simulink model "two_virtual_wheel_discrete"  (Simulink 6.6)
settings: Solver=FixedStepDiscrete  SolverMode=MultiTasking  StartTime=0.0  StopTime=tfinal  RelTol=1e-3
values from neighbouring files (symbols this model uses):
  b1 = T1*k1    (= 0.15)    [two_virtual_wheel_params.m]    (also in two_virtual_wheels.m)
  b2 = T2*k2    (= 0.015)    [two_virtual_wheel_params.m]    (also in two_virtual_wheels.m)
  Jw1 = .5*1.5/4    (= 0.1875)    [two_virtual_wheel_params.m]    (also in two_virtual_wheels.m)
  Jw2 = .5*.015/4    (= 0.001875)    [two_virtual_wheel_params.m]    (also in two_virtual_wheels.m)
  k1 = .5*15    (= 7.5)    [two_virtual_wheel_params.m]    (also in two_virtual_wheels.m)
  k2 = .5*15    (= 7.5)    [two_virtual_wheel_params.m]    (also in two_virtual_wheels.m)
  step_time = 1    [two_virtual_wheel_params.m]    (also in two_virtual_wheels.m)
  T1 = 1/50    (= 0.02)    [two_virtual_wheel_params.m]    (also in two_virtual_wheels.m)
  T2 = 1/500    (= 0.002)    [two_virtual_wheel_params.m]    (also in two_virtual_wheels.m)
  Theta_z_0 = 45    [two_virtual_wheel_params.m]    (also in two_virtual_wheels.m)
undefined symbols (not defined in the file or in its folder): DiscIntNeverNeededParam

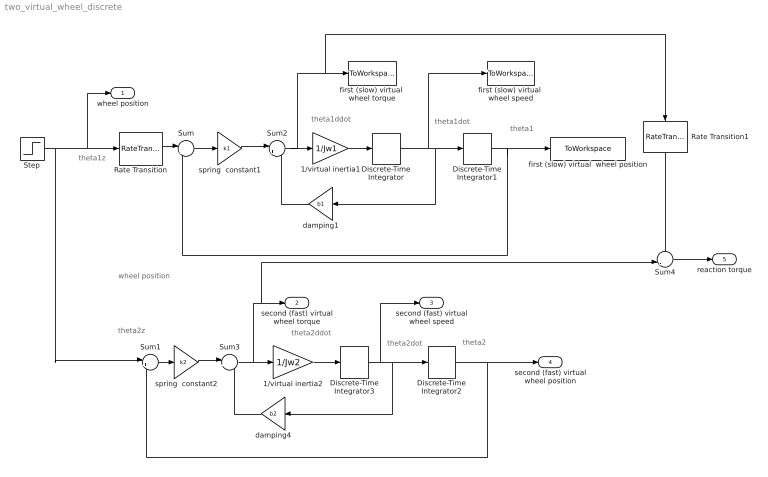
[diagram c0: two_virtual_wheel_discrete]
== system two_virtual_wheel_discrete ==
  note: theta1
  note: theta1dot
  note: theta1ddot
  note: theta1z
  note: theta2
  note: theta2dot
  note: theta2ddot
  note: theta2z
  note: wheel position
  1/virtual inertia1 : Gain  Gain=1/Jw1
  1/virtual inertia2 : Gain  Gain=1/Jw2
  Discrete-Time Integrator : DiscreteIntegrator  SampleTime=T1  ICPrevOutput=DiscIntNeverNeededParam  ICPrevScaledInput=DiscIntNeverNeededParam
  Discrete-Time Integrator1 : DiscreteIntegrator  SampleTime=T1  ICPrevOutput=DiscIntNeverNeededParam  ICPrevScaledInput=DiscIntNeverNeededParam
  Discrete-Time Integrator2 : DiscreteIntegrator  SampleTime=T2  ICPrevOutput=DiscIntNeverNeededParam  ICPrevScaledInput=DiscIntNeverNeededParam
  Discrete-Time Integrator3 : DiscreteIntegrator  SampleTime=T2  ICPrevOutput=DiscIntNeverNeededParam  ICPrevScaledInput=DiscIntNeverNeededParam
  Rate Transition : RateTransition
  Rate Transition1 : RateTransition  Orientation=down
  Step : Step  Time=step_time  After=Theta_z_0  SampleTime=T2
  Sum{,1..3} (4 alike) : Sum  Inputs=|+-
  Sum4 : Sum  Inputs=-|-
  damping1 : Gain  Orientation=left  Gain=b1
  damping4 : Gain  Orientation=left  Gain=b2
  first (slow) virtual  wheel position : ToWorkspace  VariableName=theta1  SampleTime=T1  SaveFormat=Structure With Time
  first (slow) virtual  wheel speed : ToWorkspace  VariableName=speed1  SampleTime=T1  SaveFormat=Structure With Time
  first (slow) virtual  wheel torque : ToWorkspace  VariableName=torque1  SampleTime=T1  SaveFormat=Structure With Time
  spring  constant1 : Gain  Gain=k1
  spring  constant2 : Gain  Gain=k2
  wheel position : Outport
  second (fast) virtual wheel torque : Outport  Port=2
  second (fast) virtual wheel speed : Outport  Port=3
  second (fast) virtual wheel position : Outport  Port=4
  reaction torque : Outport  Port=5
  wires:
  Discrete-Time Integrator1/1 -> Sum/2, first (slow) virtual  wheel position/1
  Sum/1 -> spring  constant1/1
  Step/1 -> wheel position/1, Rate Transition/1, Sum1/1
  1/virtual inertia1/1 -> Discrete-Time Integrator/1
  Discrete-Time Integrator/1 -> Discrete-Time Integrator1/1, damping1/1, first (slow) virtual  wheel speed/1
  Discrete-Time Integrator2/1 -> Sum1/2, second (fast) virtual wheel position/1
  Sum1/1 -> spring  constant2/1
  1/virtual inertia2/1 -> Discrete-Time Integrator3/1
  Discrete-Time Integrator3/1 -> Discrete-Time Integrator2/1, damping4/1, second (fast) virtual wheel speed/1
  Rate Transition/1 -> Sum/1
  spring  constant1/1 -> Sum2/1
  Sum2/1 -> 1/virtual inertia1/1, first (slow) virtual  wheel torque/1, Rate Transition1/1
  damping1/1 -> Sum2/2
  Sum3/1 -> 1/virtual inertia2/1, second (fast) virtual wheel torque/1, Sum4/2
  damping4/1 -> Sum3/2
  spring  constant2/1 -> Sum3/1
  Rate Transition1/1 -> Sum4/1
  Sum4/1 -> reaction torque/1
